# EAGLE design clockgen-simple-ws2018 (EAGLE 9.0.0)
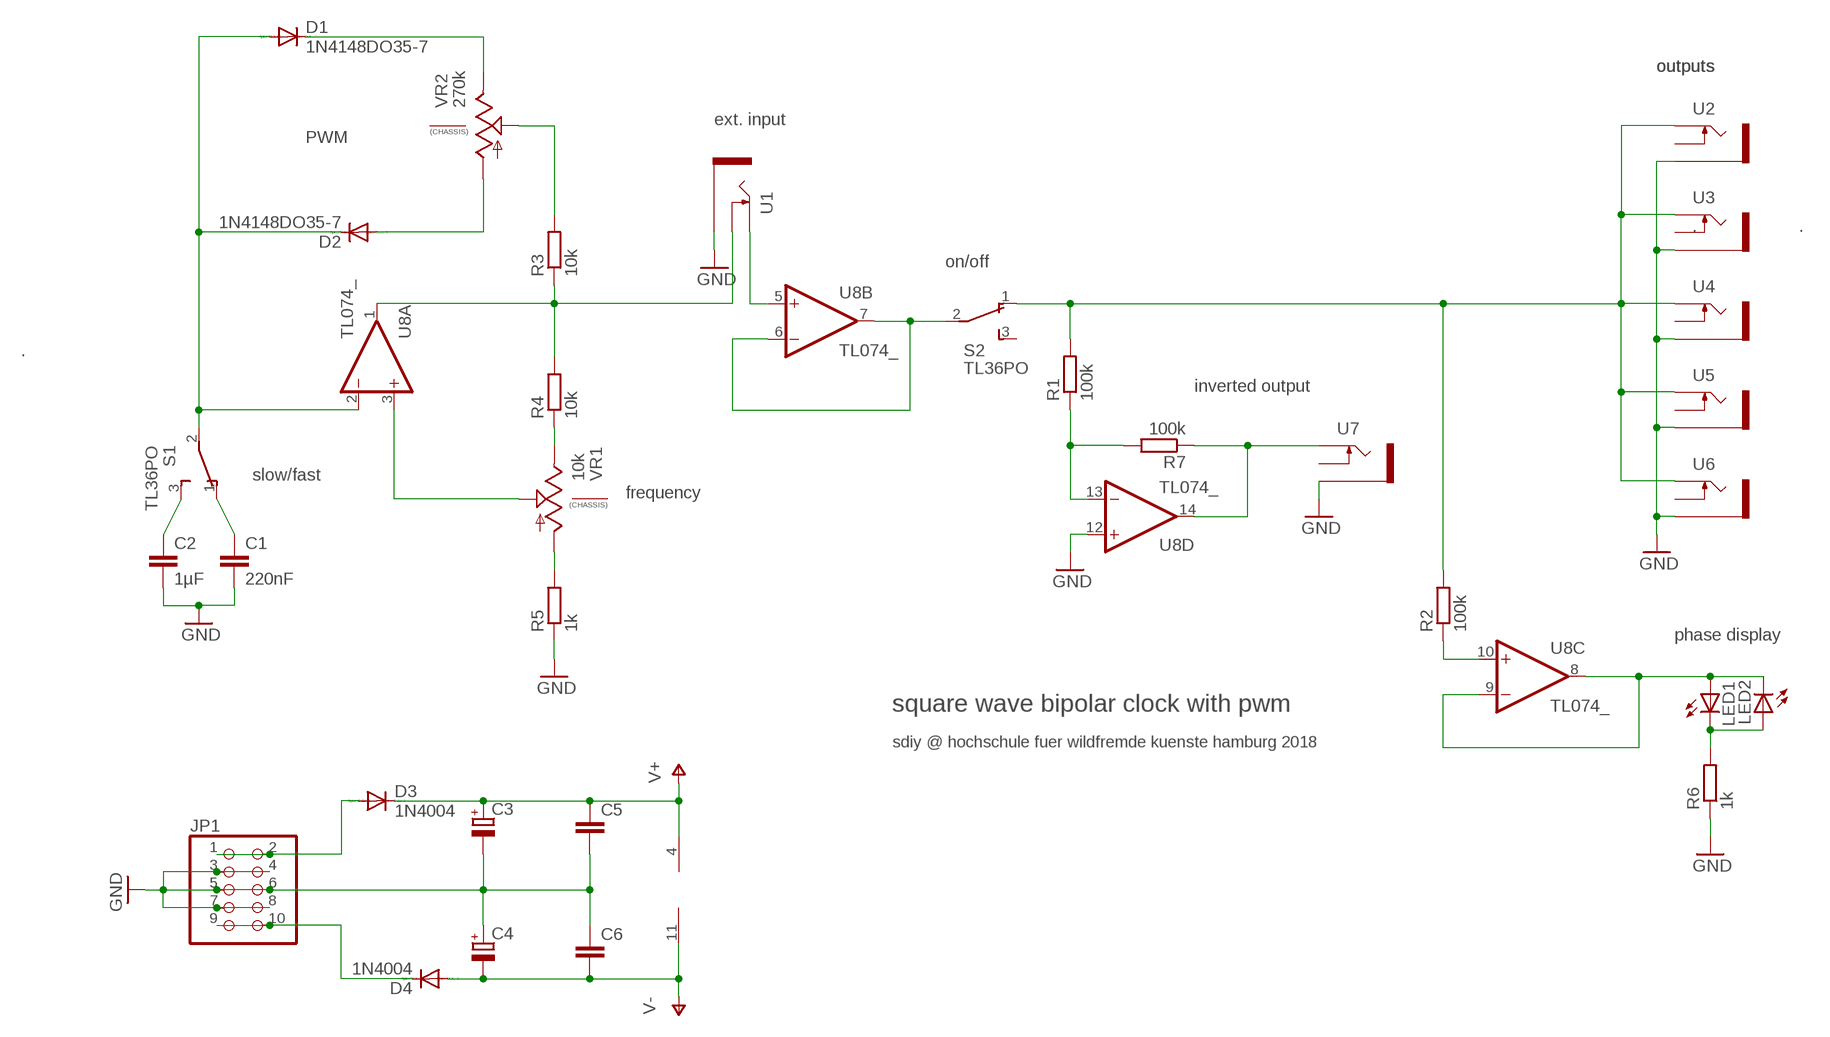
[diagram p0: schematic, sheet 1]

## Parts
C1  220nF  C-EU025-025X050  [C025-025X050]
C2  1µF  C-EU025-040X050  [C025-040X050]
C3  CPOL-EUE2.5-5  [E2,5-5]
C4  CPOL-EUE2.5-5  [E2,5-5]
C5  C-EU025-024X044  [C025-024X044]
C6  C-EU025-024X044  [C025-024X044]
D1  1N4148DO35-7  [DO35-7]
D2  1N4148DO35-7  [DO35-7]
D3  1N4004  [DO41-10]
D4  1N4004  [DO41-10]
JP1  PINHD-2X5  [2X05]
LED1  LED3MM  [LED3MM]
LED2  LED3MM  [LED3MM]
R1  100k  R-EU_0204/5  [0204/5]
R2  100k  R-EU_0204/5  [0204/5]
R3  10k  R-EU_0204/5  [0204/5]
R4  10k  R-EU_0204/5  [0204/5]
R5  1k  R-EU_0204/5  [0204/5]
R6  1k  R-EU_0204/5  [0204/5]
R7  100k  R-EU_0204/5  [0204/5]
S1  TL36PO  [TL3XPO]
S2  TL36PO  [TL3XPO]
U1  THONKICONNOLD  [THONKICONN]
U2  THONKICONNOLD  [THONKICONN]
U3  THONKICONNOLD  [THONKICONN]
U4  THONKICONNOLD  [THONKICONN]
U5  THONKICONNOLD  [THONKICONN]
U6  THONKICONNOLD  [THONKICONN]
U7  THONKICONNOLD  [THONKICONN]
U8  TL074_  [DIL14]
VR1  10k  9MM_SNAP-IN_POT_CHASSIS  [9MM_SNAP-IN_POT]
VR2  270k  9MM_SNAP-IN_POT_CHASSIS  [9MM_SNAP-IN_POT]

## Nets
GND: C1.2 C2.2 C3.- C4.+ C5.2 C6.1 JP1.3 JP1.4 JP1.5 JP1.6 JP1.7 JP1.8 R5.1 R6.1 U1.P$1_SLEEVE(SLEEVE) U2.P$1_SLEEVE(SLEEVE) U3.P$1_SLEEVE(SLEEVE) U4.P$1_SLEEVE(SLEEVE) U5.P$1_SLEEVE(SLEEVE) U6.P$1_SLEEVE(SLEEVE) U7.P$1_SLEEVE(SLEEVE) U8.12(D:+IN)
N$1: R3.2 VR2.2(S)
N$2: C1.1 S1.1(O)
N$3: C2.1 S1.3(S)
N$4: R4.1 VR1.3(E)
N$5: R5.2 VR1.1(A)
N$6: R1.2 R2.2 S2.1(O) U2.P$3_TIP(TIP) U3.P$3_TIP(TIP) U4.P$3_TIP(TIP) U5.P$3_TIP(TIP) U6.P$3_TIP(TIP)
N$7: D1.C VR2.3(E)
N$8: D2.A VR2.1(A)
N$9: D1.A D2.C S1.2(P) U8.2(A:-IN)
N$10: R3.1 R4.2 U1.P$2_SWITCH(SWITCH) U8.1(A:OUT)
N$11: S2.2(P) U8.6(B:-IN) U8.7(B:OUT)
N$12: U8.3(A:+IN) VR1.2(S)
N$13: U1.P$3_TIP(TIP) U8.5(B:+IN)
N$14: D3.A JP1.1 JP1.2
N$15: D4.C JP1.9 JP1.10
N$16: R7.1 U7.P$3_TIP(TIP) U8.14(D:OUT)
N$17: LED1.A LED2.K(C) U8.8(C:OUT) U8.9(C:-IN)
N$18: LED1.K(C) LED2.A R6.2
N$19: R2.1 U8.10(C:+IN)
N$20: R1.1 R7.2 U8.13(D:-IN)
V+: C3.+ C5.1 D3.C U8.4(P:V+)
V-: C4.- C6.2 D4.A U8.11(P:V-)
Unconnected: S2.3(S) U2.P$2_SWITCH(SWITCH) U3.P$2_SWITCH(SWITCH) U4.P$2_SWITCH(SWITCH) U5.P$2_SWITCH(SWITCH) U6.P$2_SWITCH(SWITCH) U7.P$2_SWITCH(SWITCH) VR1.CHASSIS1 VR1.CHASSIS2 VR2.CHASSIS1 VR2.CHASSIS2

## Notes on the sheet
- outputs | outputs
- ext. input
- PWM
- . | .
- on/off
- .
- inverted output
- slow/fast
- frequency
- phase display
- square wave bipolar clock with pwm
- sdiy @ hochschule fuer wildfremde kuenste hamburg 2018

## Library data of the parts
C1 C2 C5 C6 = rcl:C-EU: CAPACITOR, European symbol
C3 C4 = resistor:CPOL-EU: POLARIZED CAPACITOR, European symbol
D1 D2 = diode:1N4148: DIODE
D3 D4 = diode:1N4004: DIODE
JP1 = pinhead:PINHD-2X5: PIN HEADER
LED1 LED2 = led:LED: LED
R1-R7 = rcl:R-EU_: RESISTOR, European symbol
S1 S2 = switch:TL36PO: TINY SWITCH ON - ON Source: http://www2.produktinfo.conrad.com/datenblaetter/700000-724999/705152-da-01-de-Subminiaturschalter_TL_36YO.pdf
U1-U7 = MusicThingModular:THONKICONN: 3.5mm socket for Eurorack modular synths
U8 = MusicThingModular:TL074: Generic Quad Op Amp
VR1 VR2 = MusicThingModular:9MM_SNAP-IN_POT_CHASSIS: 9mm vertical snap-in pot, Alpha / Panasonic style, with a connection to the metal chassis for grounding

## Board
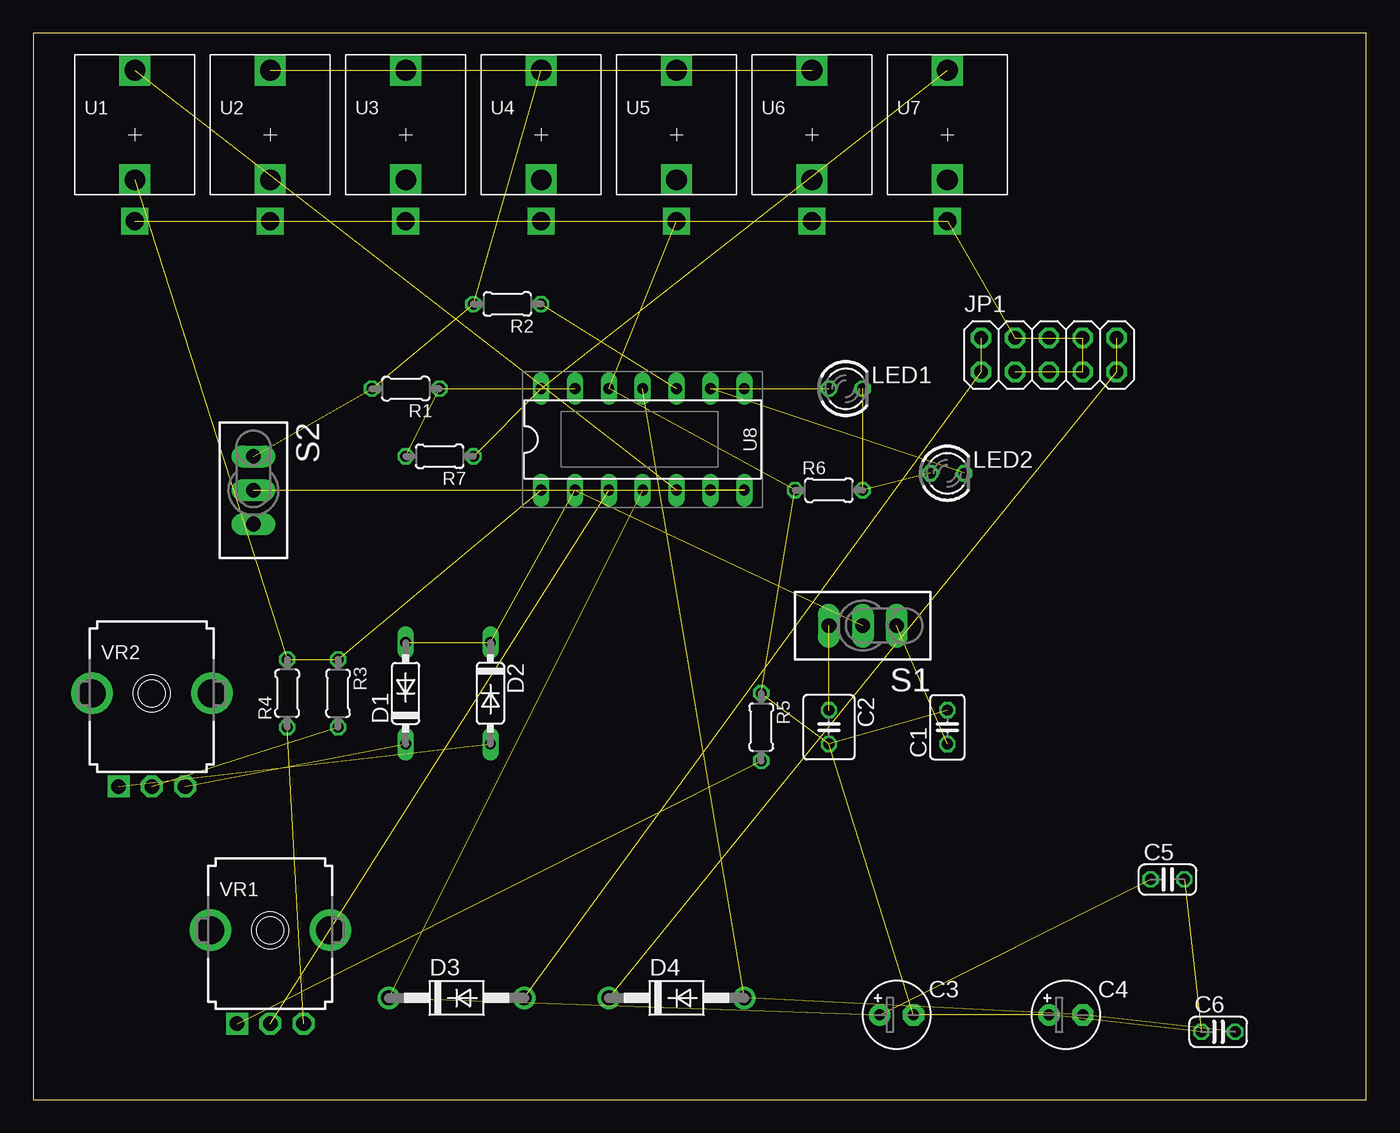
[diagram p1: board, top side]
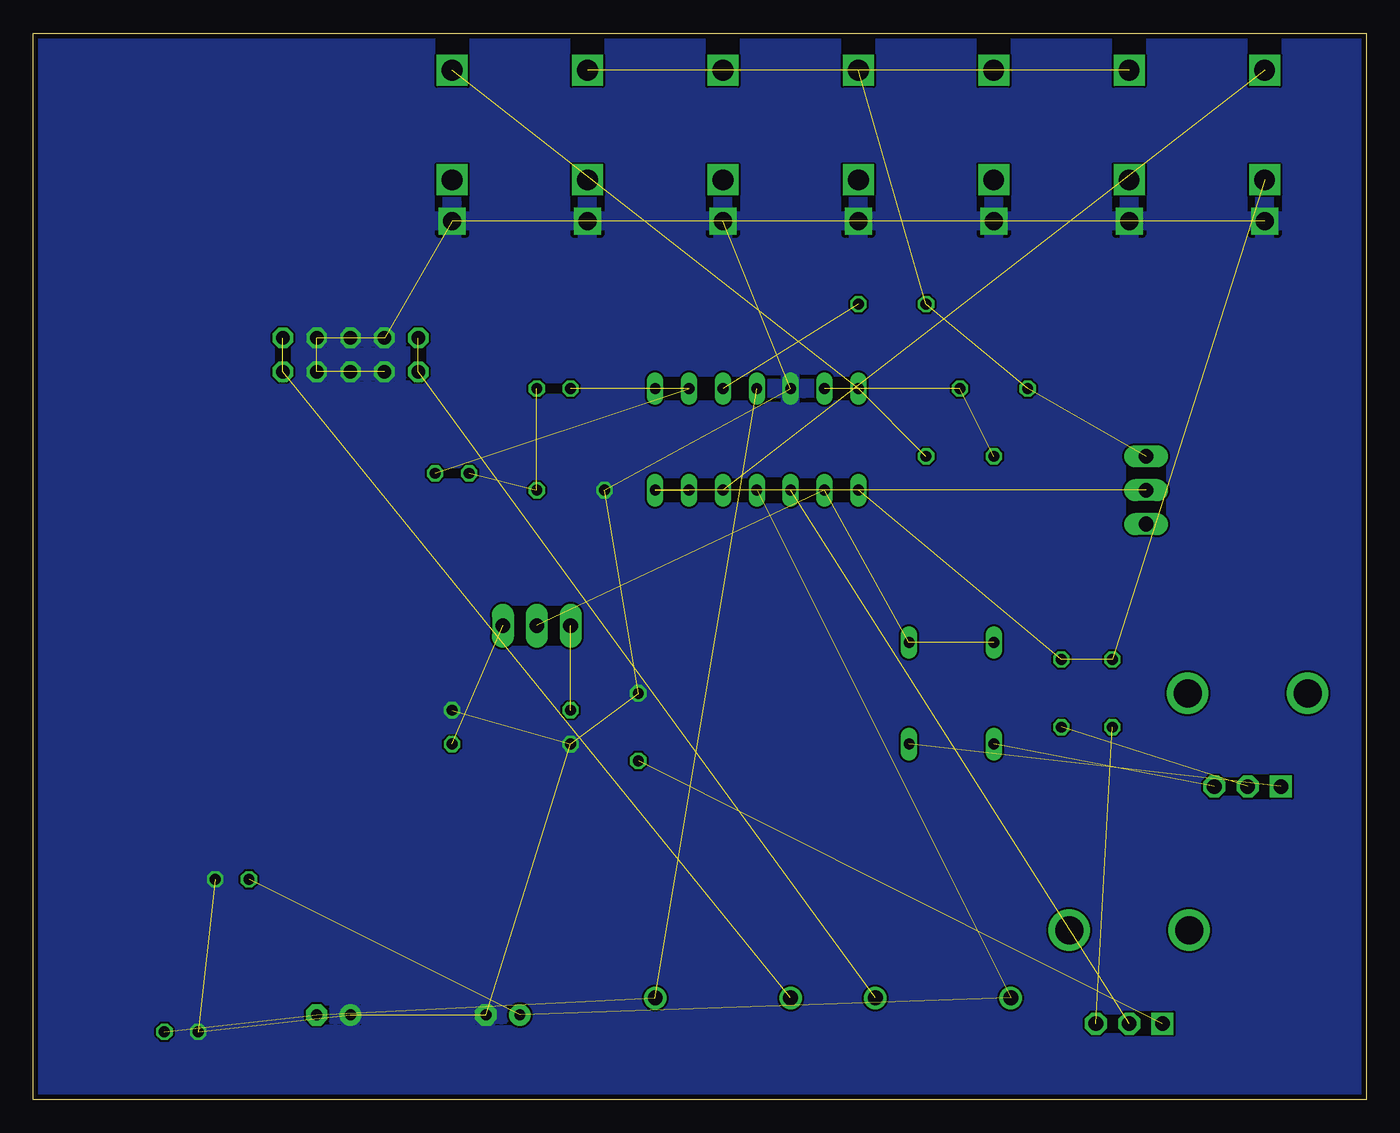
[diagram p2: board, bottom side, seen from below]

Size 100 x 80 mm. Coordinates in mm from the lower left corner, seen from the top.
Outline: 0,0 100,0 100,80 0,80 0,0
Copper layers (1*16): Top 0.0356mm / dielectric 1.5011mm / Bottom 0.0356mm
Design rules "default": minimum track width 6mil, minimum drill 13mil, track to track 6mil, track to pad 6mil, pad to pad 6mil, via to via 6mil, smd to smd 6mil, copper to edge 15mil, drill to drill 6mil, minimum pad ring 7mil, minimum via ring 7mil, stop-mask expansion 4mil, vias tented up to drill 0mil, thermal gap 10mil

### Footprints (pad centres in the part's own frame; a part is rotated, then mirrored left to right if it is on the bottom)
C025-025X050 = drill 0.813 octagon: 1 -1.27,0; 2 1.27,0
C025-040X050 = drill 0.813 octagon: 1 -1.27,0; 2 1.27,0
E2,5-5 = drill 0.813 pad 1.6: + -1.27,0 | drill 0.813 pad 1.6 octagon: - 1.27,0
C025-024X044 = drill 0.813 octagon: 1 -1.27,0; 2 1.27,0
DO35-7 = drill 0.813 long: A 3.81,0; C -3.81,0
DO41-10 = drill 1.118: A 5.08,0; C -5.08,0
2X05 = drill 1.016 octagon: 1 -5.08,-1.27; 2 -5.08,1.27; 3 -2.54,-1.27; 4 -2.54,1.27; 5 0,-1.27; 6 0,1.27; 7 2.54,-1.27; 8 2.54,1.27; 9 5.08,-1.27; 10 5.08,1.27
LED3MM = drill 0.813 octagon: A -1.27,0; K 1.27,0
0204/5 = drill 0.813 octagon: 1 -2.54,0; 2 2.54,0
TL3XPO = drill 1.1 pad 1.422 long: 1 -2.54,0; 2 0,0; 3 2.54,0
THONKICONN = drill 1.35 square: P$1_SLEEVE 0,-6.48 | drill 1.55 square: P$2_SWITCH 0,-3.38; P$3_TIP 0,4.84
DIL14 = drill 0.813 long: 1 -7.62,-3.81; 2 -5.08,-3.81; 3 -2.54,-3.81; 4 0,-3.81; 5 2.54,-3.81; 6 5.08,-3.81; 7 7.62,-3.81; 8 7.62,3.81; 9 5.08,3.81; 10 2.54,3.81; 11 0,3.81; 12 -2.54,3.81; 13 -5.08,3.81; 14 -7.62,3.81
9MM_SNAP-IN_POT = drill 1.1 square: 1 -2.5,-7 | drill 1.1 octagon: 2 0,-7; 3 2.5,-7 | drill 2.1 pad 2.794: CHASSIS1 -4.5,0; CHASSIS2 4.5,0

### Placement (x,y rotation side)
C1  68.58,27.94 90 top
C2  59.69,27.94 270 top
C3  64.77,6.35 0 top
C4  77.47,6.35 0 top
C5  85.09,16.51 0 top
C6  88.9,5.08 0 top
D1  27.94,30.48 90 top
D2  34.29,30.48 270 top
D3  31.75,7.62 0 top
D4  48.26,7.62 0 top
JP1  76.2,55.88 0 top
LED1  60.96,53.34 0 top
LED2  68.58,46.99 0 top
R1  27.94,53.34 180 top
R2  35.56,59.69 180 top
R3  22.86,30.48 270 top
R4  19.05,30.48 90 top
R5  54.61,27.94 270 top
R6  59.69,45.72 0 top
R7  30.48,48.26 180 top
S1  62.23,35.56 180 top
S2  16.51,45.72 270 top
U1  7.62,72.39 0 top
U2  17.78,72.39 0 top
U3  27.94,72.39 0 top
U4  38.1,72.39 0 top
U5  48.26,72.39 0 top
U6  58.42,72.39 0 top
U7  68.58,72.39 0 top
U8  45.72,49.53 0 top
VR1  17.78,12.7 0 top
VR2  8.89,30.48 0 top

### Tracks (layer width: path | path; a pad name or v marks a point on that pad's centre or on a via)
GND  (21 unrouted)
  pour Bottom: 0,80.01 100.33,80.01 100.33,0 0,0
N$1  (1 unrouted)
N$2  (1 unrouted)
N$3  (1 unrouted)
N$4  (1 unrouted)
N$5  (1 unrouted)
N$6  (7 unrouted)
N$7  (1 unrouted)
N$8  (1 unrouted)
N$9  (3 unrouted)
N$10  (3 unrouted)
N$11  (2 unrouted)
N$12  (1 unrouted)
N$13  (1 unrouted)
N$14  (2 unrouted)
N$15  (2 unrouted)
N$16  (2 unrouted)
N$17  (3 unrouted)
N$18  (2 unrouted)
N$19  (1 unrouted)
N$20  (2 unrouted)
V+  (3 unrouted)
V-  (3 unrouted)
